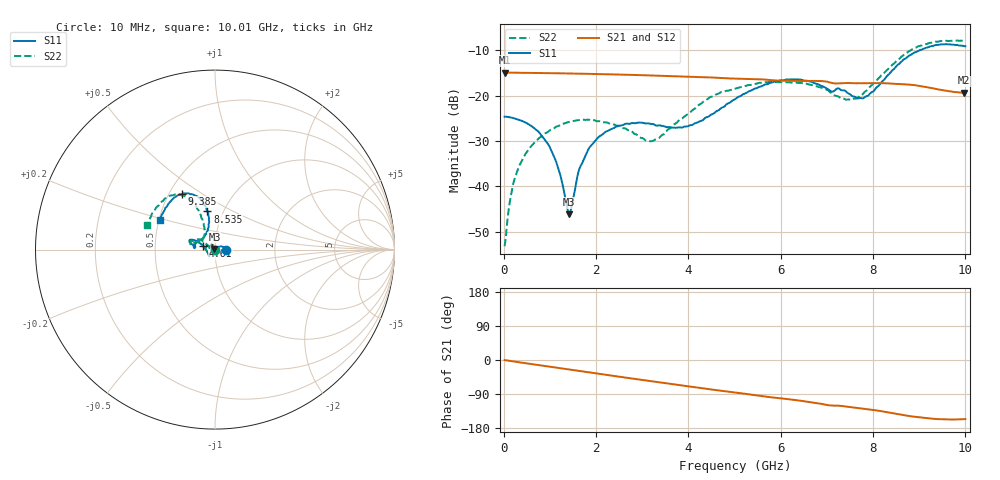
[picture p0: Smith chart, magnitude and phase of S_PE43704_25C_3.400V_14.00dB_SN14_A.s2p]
! Device ID: PE43704
! Dir: z:\PE43704\PE43704_Char_1_20130516\PE43704\AMB\3p400V\14p00dB
! Serial: 14
! Insertion: A
! Impedance: 50 ohm
! Temp: Amb
! VDD: 3.400V
! Attenuation Step: 14.00dB
! IDD: 1.139731e-01mA
#  Hz  S  RI  R  50
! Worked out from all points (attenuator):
!   401 points, 10 MHz to 10.01 GHz, reference 50 ohm
!   highest |S21| = -14.93 dB at 10 MHz (marker M1); lowest = -19.4 dB at 9.985 GHz (marker M2)
!   lowest |S11| = -46.2 dB at 1.41 GHz (marker M3), VSWR 1.01, Z = 49.7 + j0.376 ohm
!   |S11| at or under -10 dB: start of sweep to 9.02 GHz
!   |S22| runs from -53.2 to -7.9 dB; largest |S21 - S12| = 0.0013
!   S11 on the Smith chart (normalised r, x): 10 MHz: 1.12, +0.00; 4.61 GHz: 0.88, +0.03; 8.535 GHz: 0.84, +0.38; 9.385 GHz: 0.58, +0.41; 10.01 GHz: 0.51, +0.19
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1e7  0.0585 0.000127  0.1794 -0.00064  0.1795 -0.000644  -0.00214 0.000493
1.85e8  0.0565 0.00571  0.1785 -0.0108  0.1785 -0.0107  -0.00239 0.00984
4.1e8  0.0506 0.0122  0.1763 -0.0239  0.1764 -0.0233  -0.00649 0.0192
9.85e8  0.0219 0.0164  0.1682 -0.0537  0.1682 -0.0537  -0.029 0.0293
1.185e9  0.00982 0.0115  0.164 -0.0639  0.1641 -0.0638  -0.0384 0.0263
1.41e9  -0.00313 0.00379  0.1585 -0.0746  0.1584 -0.0746  -0.0469 0.0208
1.685e9  -0.0162 -0.00725  0.1507 -0.0872  0.1508 -0.0871  -0.0531 0.0116
2.26e9  -0.0292 -0.0289  0.1314 -0.1103  0.1315 -0.1103  -0.0498 -0.00269
3.11e9  -0.0327 -0.0371  0.0969 -0.1361  0.097 -0.136  -0.0313 0.00508
3.36e9  -0.0343 -0.0322  0.0858 -0.1414  0.086 -0.1414  -0.0314 0.0131
3.935e9  -0.0442 -0.0112  0.0596 -0.1504  0.0598 -0.1505  -0.0506 0.032
4.61e9  -0.065 0.0186  0.0284 -0.1547  0.0289 -0.1546  -0.0868 0.0558
5.01e9  -0.0841 0.0356  0.0114 -0.1534  0.0115 -0.1534  -0.1074 0.0516
5.935e9  -0.1333 0.0554  -0.0259 -0.1438  -0.0255 -0.1441  -0.1344 0.041
6.685e9  -0.1365 0.0353  -0.0537 -0.1347  -0.0536 -0.1345  -0.1264 0.0331
7.585e9  -0.0814 0.0537  -0.0794 -0.1116  -0.0795 -0.1115  -0.064 0.0663
7.86e9  -0.0552 0.0815  -0.0867 -0.1056  -0.0867 -0.1059  -0.0576 0.097
8.36e9  -0.0336 0.1705  -0.1024 -0.0893  -0.1022 -0.0895  -0.0776 0.1864
8.535e9  -0.0424 0.2125  -0.1068 -0.0817  -0.1064 -0.0821  -0.098 0.2257
9.385e9  -0.1837 0.3103  -0.1075 -0.0486  -0.1078 -0.0482  -0.2594 0.2935
9.985e9  -0.3021 0.1767  -0.098 -0.0435  -0.0981 -0.0433  -0.3722 0.1453
1.001e10  -0.307 0.1667  -0.0981 -0.0442  -0.0986 -0.0446  -0.3764 0.1366
